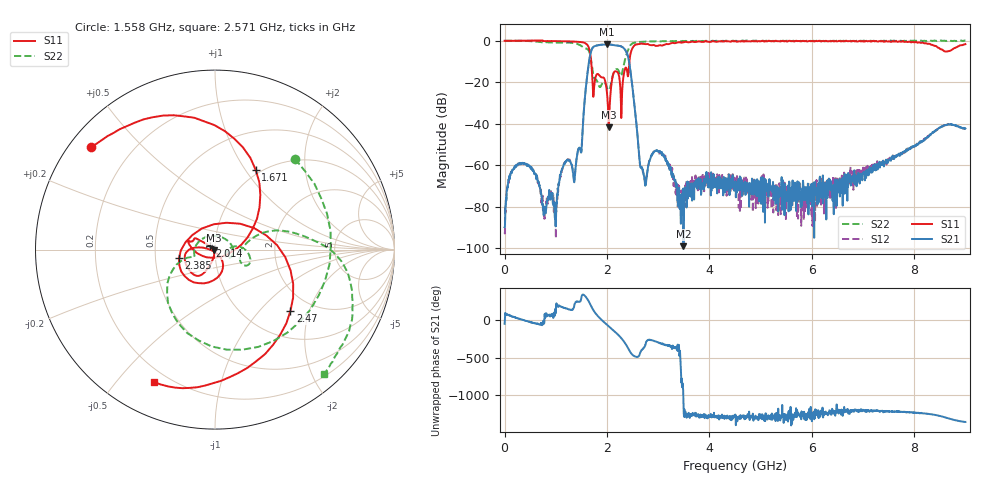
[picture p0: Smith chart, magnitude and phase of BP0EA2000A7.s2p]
!Agilent Technologies,E8358A,US40260310,A.06.04.32
!Agilent E8358A: A.06.04.32
!Date: Friday, May 08, 2020 03:29:53
!Correction: S11(Full 2 Port(1,2)) S21(Full 2 Port(1,2)) S12(Full 2 Port(1,2)) S22(Full 2 Port(1,2))
!S2P File: Measurements: S11, S21, S12, S22:
# Hz S  dB  R 50
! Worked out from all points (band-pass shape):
!   1601 points, 300 kHz to 9 GHz, reference 50 ohm
!   highest |S21| = -1.82 dB at 1.997 GHz (marker M1); lowest = -99.0 dB at 3.493 GHz (marker M2)
!   |S21| within 3 dB of the highest: 1.692 GHz to 2.365 GHz (672.8 MHz wide, 33.2 % of centre)
!   lowest |S11| = -41.8 dB at 2.036 GHz (marker M3), VSWR 1.02, Z = 49.3 - j0.424 ohm
!   |S11| at or under -10 dB: 1.69 GHz to 2.438 GHz (747.8 MHz wide, 36.2 % of centre)
!   |S22| runs from -23.8 to 0.1 dB; largest |S21 - S12| = 0.0063
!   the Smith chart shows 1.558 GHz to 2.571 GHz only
!   S11 on the Smith chart (normalised r, x): 1.558 GHz: 0.06, +0.36; 1.671 GHz: 0.94, +1.12; 2.014 GHz: 0.95, +0.03; 2.385 GHz: 0.66, -0.07; 2.47 GHz: 1.56, -1.51; 2.571 GHz: 0.15, -0.63
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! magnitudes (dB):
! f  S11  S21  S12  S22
! 300 kHz  0.0  -89.9  -92.5  0.0
! 343.4 MHz  0.0  -58.9  -58.9  -0.1
! 984.6 MHz  -0.2  -85.7  -83.9  -0.9
! 1.142 GHz  -0.3  -60.7  -60.5  -0.9
! 1.502 GHz  -0.7  -53.0  -52.9  -2.5
! 1.558 GHz  -1.0  -30.4  -30.4  -3.4
! 1.671 GHz  -6.0  -6.9  -7.0  -6.8
! 1.997 GHz  -24.5  -1.8  -1.8  -22.4
! 2.014 GHz  -29.6  -1.8  -1.8  -23.3
! 2.036 GHz  -41.8  -1.8  -1.8  -23.8
! 2.143 GHz  -15.0  -2.1  -2.1  -14.8
! 2.278 GHz  -37.3  -2.8  -2.7  -16.8
! 2.385 GHz  -13.7  -5.8  -5.7  -6.3
! 2.47 GHz  -5.3  -16.8  -16.8  -1.8
! 2.571 GHz  -1.8  -39.2  -39.1  -0.7
! 2.734 GHz  -1.6  -66.0  -66.9  -0.5
! 3.004 GHz  -2.4  -53.3  -53.4  -0.3
! 3.493 GHz  -0.8  -99.0  -72.3  -0.2
! 4.5 GHz  -0.2  -70.9  -69.1  -0.1
! 6.002 GHz  -0.1  -79.7  -69.0  -0.2
! 7.504 GHz  -0.3  -57.7  -57.2  -0.1
! 9 GHz  -1.6  -42.3  -42.7  0.0
